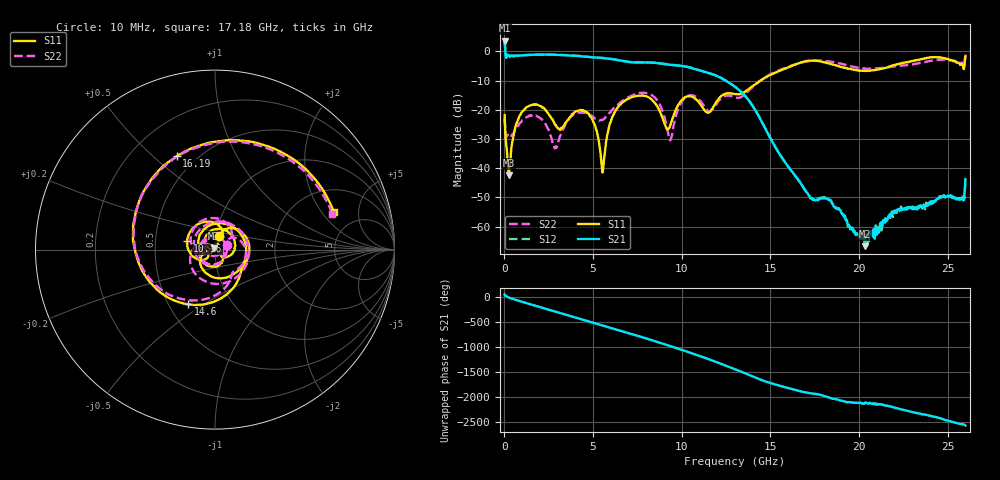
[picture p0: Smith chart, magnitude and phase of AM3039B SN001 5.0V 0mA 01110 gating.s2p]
!Agilent Technologies,E8364B,MY43040894,A.07.50.67
!Agilent E8364B: A.07.50.67
!Date: Tuesday, June 28, 2016 08:06:42
!Correction: S11(Full 2 Port(1,2))
!S21(Full 2 Port(1,2))
!S12(Full 2 Port(1,2))
!S22(Full 2 Port(1,2))
!S2P File: Measurements: S11, S21, S12, S22:
# Hz S  dB  R 50
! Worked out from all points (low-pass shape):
!   1601 points, 10 MHz to 26 GHz, reference 50 ohm
!   highest |S21| = 3.70 dB at 10 MHz (marker M1); lowest = -66.7 dB at 20.33 GHz (marker M2)
!   |S21| within 3 dB of the highest: start of sweep to 44.15 MHz
!   lowest |S11| = -42.5 dB at 253.7 MHz (marker M3), VSWR 1.02, Z = 49.6 + j0.621 ohm
!   |S11| at or under -10 dB: start of sweep to 14.44 GHz
!   |S22| runs from -33.3 to -1.1 dB; largest |S21 - S12| = 0.025
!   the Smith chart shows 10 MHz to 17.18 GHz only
!   S11 on the Smith chart (normalised r, x): 10 MHz: 1.03, +0.16; 10.16 GHz: 0.73, +0.07; 14.6 GHz: 0.63, -0.43; 16.19 GHz: 0.39, +0.60; 17.18 GHz: 3.25, +2.65
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1e7  -21.86 74.7  3.70 40.9  3.76 41.7  -23.11 21.7
2.536562e8  -42.49 123.5  -1.37 -18.7  -1.32 -18.4  -29.02 -60.7
1.634375e9  -18.12 56.0  -1.14 -169.8  -1.09 -169.6  -21.61 59.8
2.657731e9  -22.97 -36.1  -1.12 85.3  -1.06 85.6  -29.79 -42.3
3.486162e9  -24.14 -43.2  -1.32 0.4  -1.27 0.6  -24.58 -37.7
4.347081e9  -20.23 -121.6  -1.67 -89.0  -1.63 -88.8  -20.89 -146.8
5.971456e9  -24.43 -161.6  -2.55 100.4  -2.49 100.5  -20.93 -117.0
6.994812e9  -16.23 67.7  -3.61 -6.6  -3.56 -6.4  -15.70 68.4
8.684162e9  -19.53 -142.0  -4.04 171.7  -3.97 171.9  -17.40 -170.9
1.016234e10  -15.78 163.2  -5.13 2.2  -5.07 2.2  -16.01 146.3
1.154306e10  -20.87 67.8  -7.45 -167.0  -7.39 -167.1  -20.54 35.2
1.3005e10  -14.62 -22.3  -12.14 -4.1  -12.10 -4.3  -15.74 -43.8
1.459689e10  -9.40 -116.0  -25.07 128.4  -25.00 128.2  -9.34 -128.1
1.618878e10  -5.01 112.3  -40.99 -35.4  -40.91 -35.4  -4.83 103.5
1.717964e10  -3.17 17.7  -49.54 -118.8  -49.28 -117.7  -3.32 17.1
1.734208e10  -3.13 1.2  -50.28 -125.6  -50.63 -125.0  -3.23 2.7
1.841417e10  -4.31 -101.7  -51.13 140.4  -51.16 142.1  -3.50 -92.6
2.033093e10  -6.65 109.8  -66.74 40.6  -63.92 25.1  -5.86 118.8
2.167916e10  -5.22 18.2  -56.34 -19.4  -57.66 -11.5  -5.37 23.7
2.315734e10  -3.07 -92.8  -53.80 -148.5  -54.41 -148.1  -4.28 -83.7
2.426192e10  -1.99 177.3  -51.42 129.9  -51.20 131.3  -3.02 -168.0
2.6e10  -1.73 -19.7  -43.84 -42.3  -43.67 -40.1  -1.05 10.0
